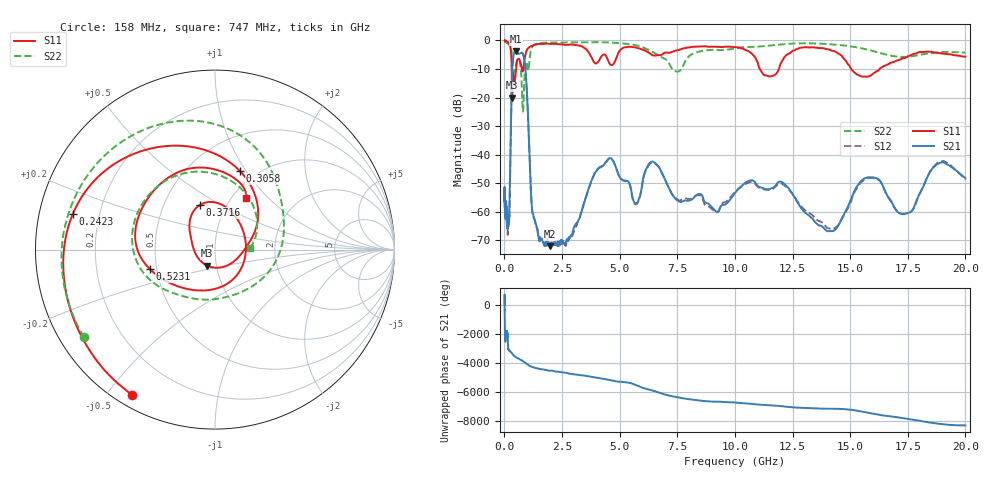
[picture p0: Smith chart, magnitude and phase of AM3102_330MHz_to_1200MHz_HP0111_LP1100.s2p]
! Date/Time: Tue, Sep 11, 2018 5:16 PM
! Network Analyzer: Agilent Technologies E8362B Rev: A.07.50.63
! Sweep from 0.010 to 20.000 GHz, 1601 Points, Sweep Type: LOG
! Power Supply: 4.949 V, 0.001 A
# Hz S DB R 50
!freq MagS11 AngS11 MagS21 AngS21 MagS12 AngS12 MagS22 AngS22
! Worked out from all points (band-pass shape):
!   1601 points, 10 MHz to 20 GHz, reference 50 ohm
!   highest |S21| = -3.82 dB at 487.1 MHz (marker M1); lowest = -72.1 dB at 1.978 GHz (marker M2)
!   |S21| within 3 dB of the highest: 366.9 MHz to 865.2 MHz (498.3 MHz wide, 80.9 % of centre)
!   lowest |S11| = -20.0 dB at 341.1 MHz (marker M3), VSWR 1.22, Z = 45.1 - j8.17 ohm
!   |S11| at or under -10 dB: 317.3 MHz to 505.5 MHz (188.2 MHz wide, 45.8 % of centre); 11.08 GHz to 11.91 GHz (830.3 MHz wide, 7.22 % of centre); 15.04 GHz to 16.28 GHz (1.238 GHz wide, 7.9 % of centre)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
!   |S22| runs from -24.9 to -0.3 dB; largest |S21 - S12| = 0.011
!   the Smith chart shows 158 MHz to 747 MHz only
!   S11 on the Smith chart (normalised r, x): 158 MHz: 0.05, -0.58; 242.3 MHz: 0.10, +0.12; 305.8 MHz: 0.84, +0.94; 371.6 MHz: 0.75, +0.40; 523.1 MHz: 0.46, -0.12; 747 MHz: 1.16, +0.75
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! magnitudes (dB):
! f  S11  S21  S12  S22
! 10 MHz  0.0  -52.2  -51.7  -0.3
! 35.55 MHz  0.0  -60.8  -59.9  -0.5
! 126.4 MHz  -0.4  -62.5  -65.4  -1.0
! 158 MHz  -0.6  -62.8  -64.9  -1.1
! 242.3 MHz  -1.8  -50.4  -51.3  -1.7
! 305.8 MHz  -6.7  -20.7  -20.7  -3.2
! 341.1 MHz  -20.0  -9.8  -9.9  -6.1
! 371.6 MHz  -11.6  -6.5  -6.6  -8.5
! 447.2 MHz  -14.6  -4.0  -4.0  -11.0
! 487.1 MHz  -11.8  -3.8  -3.9  -9.6
! 523.1 MHz  -8.4  -4.1  -4.2  -7.8
! 747 MHz  -9.5  -4.3  -4.3  -14.2
! 942.8 MHz  -4.1  -13.4  -13.5  -7.6
! 1.213 GHz  -1.8  -59.8  -60.2  -2.2
! 1.59 GHz  -1.3  -69.5  -69.8  -0.9
! 1.978 GHz  -1.2  -72.1  -71.1  -0.8
! 2.746 GHz  -1.5  -69.7  -70.5  -0.7
! 4.521 GHz  -7.5  -41.5  -41.4  -0.7
! 5.652 GHz  -2.4  -56.9  -57.3  -1.6
! 6.487 GHz  -5.3  -42.6  -43.0  -4.2
! 14.01 GHz  -3.1  -66.8  -65.7  -1.3
! 20 GHz  -5.7  -48.2  -48.8  -4.2
